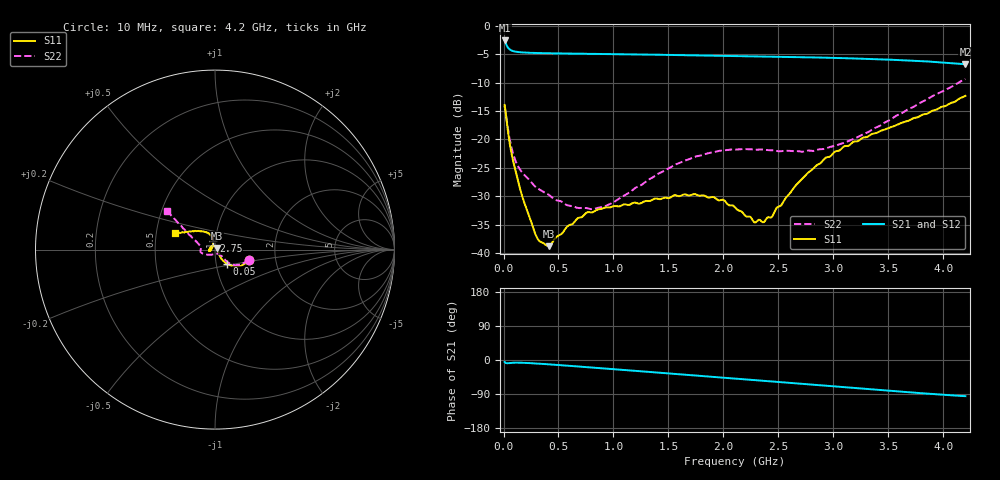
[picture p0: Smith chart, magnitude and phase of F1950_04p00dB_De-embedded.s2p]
! Integrated Device Technology
! Corporate Headquarters
! 6024 Silver Creek Valley Road
! San Jose, CA 95138  USA
! Phone:  1-408-284-8200
! Toll Free:  1-800-223-1366
! Webpage:  http://www.idt.com/
! Timing and RF Division
! 515 Groton Road, Suite 102
! Westford, MA 01886-6024
! Device:  F1950
! Description: 7-bit 0.25 dB Digital Step Attenuator
! Frequency:  150.0 -  4000.00 MHz
! Package:  4x4 mm Thin QFN Plastic Package: 24 pin
! Ports:  2 RF, 12 DC
!  Pin  1  = D0
!  Pin  2  = VDD
!  Pin  3  = Vmode
!  Pin  4  = GND
!  Pin  5  = RF1  =  Port 1
!  Pin  6  = GND
!  Pin  7  = GND
!  Pin  8  = GND
!  Pin  9  = GND
!  Pin 10  = GND
!  Pin 11  = GND
!  Pin 12  = GND
!  Pin 13  = GND
!  Pin 14  = RF2  =  Port 2
!  Pin 15  = GND
!  Pin 16  = LE
!  Pin 17  = CLK
!  Pin 18  = DATE
!  Pin 19  = D6
!  Pin 20  = D5
!  Pin 21  = D4
!  Pin 22  = D3
!  Pin 23  = D2
!  Pin 24  = D1
! State:  16
! Atten State:  4.00 dB
! Voltage:  +5.00 Volts
! Current:  Not Measured mA
! Data:  The device was measured on a the F195X evaluation board which has
!  individual transmission lines to the RF pins.  Data was collected
!  using a calibrated network analyzer.  The evaluation board was
!  de-embedded using a TRL calibration technique.
!  The reference plane is the edge of the package pin.
! Misc:  Board 2019
!  Action Tracker AT0250
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# GHz S dB R 50
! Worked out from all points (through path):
!   420 points, 10 MHz to 4.2 GHz, reference 50 ohm
!   highest |S21| = -2.61 dB at 10 MHz (marker M1); lowest = -6.8 dB at 4.2 GHz (marker M2)
!   group delay of S21, straight-line fit = 62 ps
!   lowest |S11| = -38.7 dB at 410 MHz (marker M3), VSWR 1.02, Z = 50.9 + j0.728 ohm
!   |S11| at or under -10 dB: start of sweep to end of sweep
!   |S22| runs from -32.2 to -9.4 dB; largest |S21 - S12| = 0.00071
!   S11 on the Smith chart (normalised r, x): 10 MHz: 1.46, -0.18; 50 MHz: 1.12, -0.18; 2.75 GHz: 0.98, +0.09; 4.2 GHz: 0.63, +0.12
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0.01  -13.93 -17.4  -2.61 -5.2  -2.60 -5.2  -14.10 -16.7
0.05  -19.88 -50.2  -4.08 -8.3  -4.08 -8.3  -19.34 -44.2
0.09  -24.00 -55.1  -4.49 -7.3  -4.49 -7.3  -22.69 -44.9
0.13  -27.08 -52.9  -4.63 -7.1  -4.63 -7.1  -24.65 -44.0
0.28  -36.09 -18.6  -4.80 -8.9  -4.80 -8.9  -28.11 -45.6
0.33  -37.91 -0.0  -4.82 -9.8  -4.82 -9.8  -28.82 -47.2
0.41  -38.74 38.2  -4.85 -11.4  -4.85 -11.4  -29.68 -48.0
0.58  -35.28 84.7  -4.90 -15.0  -4.90 -15.0  -31.55 -57.4
0.71  -33.65 102.7  -4.94 -17.8  -4.94 -17.8  -32.02 -70.4
0.93  -31.94 124.2  -4.99 -22.7  -4.99 -22.7  -31.68 -98.1
1.41  -30.47 171.4  -5.12 -33.4  -5.11 -33.4  -25.98 -145.8
1.74  -29.60 -168.2  -5.21 -40.8  -5.21 -40.8  -23.04 -160.8
2  -30.61 -166.1  -5.29 -46.7  -5.29 -46.8  -21.91 -168.7
2.11  -32.00 -169.1  -5.33 -49.2  -5.32 -49.3  -21.77 -171.5
2.28  -34.53 167.0  -5.38 -53.0  -5.38 -53.1  -21.78 -175.1
2.37  -34.48 145.3  -5.42 -55.1  -5.41 -55.1  -21.77 -177.1
2.44  -33.61 129.2  -5.44 -56.6  -5.44 -56.6  -21.89 -178.8
2.75  -26.19 101.8  -5.55 -63.8  -5.55 -63.8  -22.02 171.8
2.81  -25.23 100.9  -5.58 -65.1  -5.57 -65.2  -22.01 170.4
3.1  -21.19 107.7  -5.72 -71.9  -5.71 -71.9  -20.56 162.5
3.51  -17.91 126.2  -5.98 -81.2  -5.97 -81.3  -16.64 151.7
4.2  -12.34 157.7  -6.80 -95.4  -6.79 -95.5  -9.38 141.2
